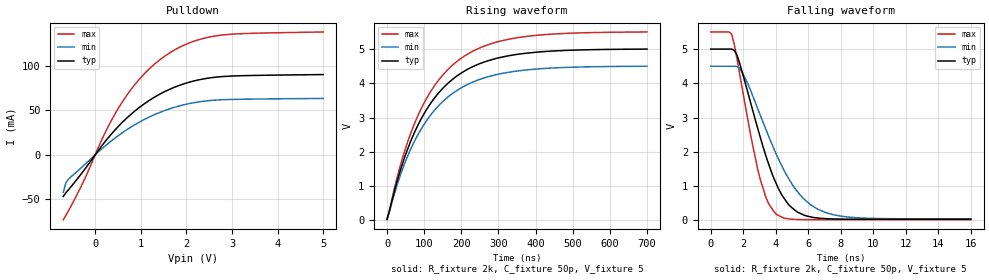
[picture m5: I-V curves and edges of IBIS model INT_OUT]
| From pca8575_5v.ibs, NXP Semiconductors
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[Model]   INT_OUT
Model_type Open_drain
Vref=5
Vmeas=2.5
Rref=2k
Cref=50p
C_comp   5.4p   5.2p   5.7p
[Temperature Range] 27   85   -40
[Voltage Range]   5   4.5   5.5
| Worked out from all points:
|   slope of the pulldown table from 0 to 0.75 V, typ, clamps not added: 17 ohm
|   falling waveform, R_fixture 2k, C_fixture 50p, V_fixture 5: 20-80 % time 1.95ns typ, 2.57ns min, 1.37ns max; typ from 5 V to 0.034 V
|   rising waveform, R_fixture 2k, C_fixture 50p, V_fixture 5: 20-80 % time 140ns typ, 140ns min, 140ns max; typ from 0.034 V to 5 V
[Pulldown]
-700mV    -46.85mA   -42.29mA   -73.04mA
-640mV    -42.51mA   -31.08mA   -67.91mA
-580mV    -38.92mA   -27.12mA   -62.44mA
-240mV    -16.96mA   -11.45mA   -28.04mA
220mV     15.08mA    10.05mA    25.19mA
510mV     32.15mA    21.75mA    52.61mA
740mV     43.6mA     29.8mA     70.39mA
970mV     53.41mA    36.83mA    85.19mA
1.49V     70.28mA    49.19mA    109.8mA
2.01V     80.97mA    57.1mA     124.9mA
2.64V     87.39mA    61.58mA    133.9mA
5V        90.34mA    63.47mA    138.3mA
[Falling Waveform]
R_fixture=2k
C_fixture=50p
V_fixture=5
V_fixture_min=4.5
V_fixture_max=5.5
0s        5V         4.5V       5.5V
1.293ns   5V         4.5V       5.431V
1.616ns   4.822V     4.492V     4.713V
1.939ns   4.321V     4.313V     3.842V
2.909ns   2.654V     3.238V     1.452V
3.394ns   1.883V     2.656V     673.6mV
4.04ns    1.064V     1.922V     178.4mV
5.333ns   243mV      844.2mV    28.27mV
7.111ns   52.14mV    223mV      22.4mV
16ns      34.47mV    47.03mV    22.34mV
[Rising Waveform]
R_fixture=2k
C_fixture=50p
V_fixture=5
V_fixture_min=4.5
V_fixture_max=5.5
0s        34.47mV    46.98mV    22.34mV
21.21ns   909.2mV    823.7mV    995.6mV
42.42ns   1.679V     1.515V     1.845V
63.64ns   2.306V     2.077V     2.536V
84.85ns   2.814V     2.533V     3.096V
134.3ns   3.659V     3.292V     4.026V
198ns     4.284V     3.855V     4.714V
268.7ns   4.644V     4.179V     5.11V
360.6ns   4.856V     4.37V      5.343V
700ns     4.995V     4.495V     5.494V
[Ramp]
R_load=2k
dV/dt_r   2.979E+0/2.094E-9   2.969E+0/2.304E-9   2.988E+0/1.868E-9
dV/dt_f   2.979E+0/9.067E-11   2.969E+0/1.508E-10   2.988E+0/6.529E-11
|[End   INT_OUT
